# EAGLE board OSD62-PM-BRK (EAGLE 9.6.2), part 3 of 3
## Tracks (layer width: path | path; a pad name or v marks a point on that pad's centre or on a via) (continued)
VIN-5P0  (via drill 0.1 pad 0.25, 0.25 pad 0.46) (continued)
  pour Bottom: 86.23,5.97 86.23,7.75 84.71,7.75 84.71,5.97
  pour Bottom (no thermals): 64.52,16.89 65.79,16.89 65.79,17.53 65.28,18.03 64.52,18.03
  pour Top (no thermals): 64.52,18.03 65.28,18.03 65.79,17.53 65.79,16.89 64.52,16.89
  pour Bottom: 5.33,10.54 5.33,11.3 4.57,11.3 4.57,10.54
VMON_ER_SYS  (via drill 0.1 pad 0.25)
  Top 0.076: U1.A15 40.26,17.25 42.6,19.58 42.6,20.42 44.2,22.02 46.02,22.02 v46.18,22.17
  Top 0.127: R1.2 45.72,24.64 | 45.72,24.64 R2.1 | v45.72,24.31 45.72,24.64
  Bottom 0.076: v46.18,22.17 46.56,22.55 46.56,24.16 46.41,24.31 v45.72,24.31
VOUT0_DATA0  (via drill 0.1 pad 0.25)
  Top 0.076: U1.P26 v46,10.5
  Bottom 0.076: v46,10.5 46.37,10.5 46.56,10.31 46.56,7.01 48.23,5.33 49.99,5.33 50.67,4.65 50.67,2.67 JP2.21
VOUT0_DATA1  (via drill 0.1 pad 0.25)
  Top 0.076: U1.N25 v45.5,11
  Bottom 0.076: v45.5,11 45.75,10.75 46.35,10.75 46.71,10.39 46.71,7.09 48.31,5.49 50.44,5.49 52.07,3.86 JP3.21
VOUT0_DATA2  (via drill 0.1 pad 0.25)
  Top 0.076: U1.N26 v46,11
  Bottom 0.076: v46,11 46.33,11 47.32,10.01 47.32,6.71 48.39,5.64 52.27,5.64 53.19,4.72 53.19,2.69 JP2.22
VOUT0_DATA3  (via drill 0.1 pad 0.25)
  Top 0.076: U1.M25 v45.5,11.5
  Bottom 0.076: v45.5,11.5 45.75,11.25 46.31,11.25 47.47,10.09 47.47,6.78 48.46,5.79 52.65,5.79 54.61,3.83 JP3.22
VOUT0_DATA4  (via drill 0.1 pad 0.25)
  Top 0.076: U1.M26 v46,11.5
  Bottom 0.076: v46,11.5 46.29,11.5 47.62,10.16 47.62,6.86 48.54,5.94 54.63,5.94 55.7,4.88 55.7,2.72 JP2.23
VOUT0_DATA5
  Top 0.076: U1.U27 46.81,8.69 48.23,8.69 52.12,4.8 56.16,4.8 JP3.23
VOUT0_DATA6
  Top 0.076: U1.T27 46.5,9.5 47.65,9.5 52.2,4.95 57.61,4.95 58.29,4.27 58.29,2.67 JP2.24
VOUT0_DATA7
  Top 0.076: U1.T28 47.63,9.75 52.27,5.11 57.68,5.11 58.45,4.34 58.45,4.04 58.67,3.81 JP3.24
VOUT0_DATA8
  Top 0.076: U1.R27 46.5,10 47.61,10 52.35,5.26 57.76,5.26 58.22,4.8 60.2,4.8 60.81,4.19 60.81,2.69 JP2.25
VOUT0_DATA9
  Top 0.076: U1.R28 47.59,10.25 52.43,5.41 57.84,5.41 58.29,4.95 61.11,4.95 62.23,3.83 JP3.25
VOUT0_DATA10
  Top 0.076: U1.P27 46.5,10.5 47.56,10.5 52.5,5.56 57.91,5.56 58.37,5.11 62.64,5.11 63.32,4.42 63.32,2.72 JP2.26
VOUT0_DATA11
  Top 0.076: U1.P28 47.54,10.75 52.58,5.71 57.99,5.71 58.45,5.26 63.32,5.26 JP3.26
VOUT0_DATA12
  Top 0.076: U1.N27 46.5,11 47.52,11 52.65,5.87 58.06,5.87 58.52,5.41 64.92,5.41 65.84,4.5 65.84,2.74 JP2.27
VOUT0_DATA13
  Top 0.076: U1.N28 47.5,11.25 52.73,6.02 58.14,6.02 58.6,5.56 65.61,5.56 67.31,3.86 JP3.27
VOUT0_DATA14
  Top 0.076: U1.M27 46.5,11.5 47.48,11.5 52.81,6.17 58.22,6.17 58.67,5.71 67.36,5.71 68.43,4.65 68.43,2.69 JP2.28
VOUT0_DATA15
  Top 0.076: U1.M28 47.46,11.75 52.88,6.33 58.29,6.33 58.75,5.87 67.82,5.87 69.85,3.83 JP3.28
VOUT0_DE  (via drill 0.1 pad 0.25)
  Top 0.076: U1.R25 v45.5,10
  Bottom 0.076: v45.5,10 45.75,9.75 45.75,9.19 45.87,9.07 45.87,2.39 JP2.19
VOUT0_HSYNC  (via drill 0.1 pad 0.25)
  Top 0.076: U1.P25 v45.5,10.5
  Bottom 0.076: v45.5,10.5 45.75,10.25 46.17,10.25 46.41,10.01 46.41,6.93 JP3.20
VOUT0_PCLK  (via drill 0.1 pad 0.25)
  Top 0.076: U1.T26 v46,9.5
  Bottom 0.076: v46,9.5 46.02,9.47 46.02,4.72 46.94,3.81 JP3.19
VOUT0_VSYNC  (via drill 0.1 pad 0.25)
  Top 0.076: U1.R26 v46,10
  Bottom 0.076: v46,10 v46.01,10 46.25,9.75 46.25,6.71 48.39,4.57 48.39,2.41 JP2.20
VPP  (via drill 0.1 pad 0.25)
  Top 0.152: U1.C16 v41,16.5
  Bottom 0.254: v41,16.5 41.15,16.65 41.15,22.99 41.6,23.44 v41.6,24.08
  pour Top (no thermals): 41.25,25.02 41.25,23.57 41.45,23.37 42.04,23.37 42.04,25.02
VPP_EN
  Top 0.076: U14.3 40.65,22.73 J1.2 38.15,23.57 R3.2
WKUP_CLKOUT0  (via drill 0.1 pad 0.25)
  Top 0.076: U1.C7 v36,16.5 | v36.04,22.78 35.89,22.63 35.89,18.14 v36.12,17.91
  Bottom 0.076: v36.12,17.91 36,17.79 v36,16.5 | v36.04,22.78 36.27,23.01 36.27,24.77 35.89,25.15 35.89,28.27 JP5.15
WKUP_I2C0_SCL  (via drill 0.1 pad 0.25)
  Top 0.076: U1.A8 36.75,17.89 36.2,18.44 36.2,22.33 37.03,23.16 37.03,25.22 37.34,25.53 43.2,25.53 v43.59,25.15 | v46.63,19.43 46.94,19.13 49.99,19.13 57.15,11.96 70.33,11.96 71.09,11.2 71.09,9.46 J4.13 71.04,8.44 71.32,8.15 76.5,8.15 76.99,8.64 R64.1
  Bottom 0.076: v46.63,19.43 47.02,19.81 47.02,24.46 46.56,24.92 43.81,24.92 v43.59,25.15
WKUP_I2C0_SDA  (via drill 0.1 pad 0.25)
  Top 0.076: U1.B8 36.5,17 36.5,17.91 36.04,18.36 36.04,22.4 36.88,23.24 36.88,25.3 37.26,25.68 43.43,25.68 v43.59,25.53 | v47.02,19.43 47.17,19.28 50.06,19.28 57.23,12.12 71.32,12.12 72.01,11.43 72.01,9.44 J4.14 72.04,8.43 72.16,8.31 76.43,8.31 77.78,9.65 R12.1
  Bottom 0.076: v47.02,19.43 47.17,19.58 47.17,24.54 46.63,25.07 44.04,25.07 v43.59,25.53
WKUP_LFOSC0_XI
  Top 0.076: U1.H1 32.88,13.75 31.09,15.54 31.09,18.44 30.94,18.59 30.11,18.59 Y1.3
WKUP_UART0_CTSN
  Top 0.076: U1.D1 32.75,15.75 32.23,16.27 32.23,21.49 31.7,22.02 25.3,22.02 22.25,25.07 20.8,25.07 20.12,25.76 20.12,27.58 19.74,27.96 17.83,27.96 17.53,28.27 16,28.27 15.06,29.21 JP5.6
WKUP_UART0_RTSN
  Top 0.076: U1.D2 33.5,16 32.75,16 32.38,16.36 32.38,21.57 31.77,22.17 25.38,22.17 22.33,25.22 20.88,25.22 20.27,25.83 20.27,27.74 19.89,28.12 18.67,28.12 17.58,29.21 JP5.7
WKUP_UART0_RXD
  Top 0.076: U1.C2 33.5,16.5 32.88,16.5 32.69,16.69 32.69,21.72 31.93,22.48 25.53,22.48 22.48,25.53 21.03,25.53 20.57,25.98 20.57,28.19 JP5.9
WKUP_UART0_TXD
  Top 0.076: U1.C1 32.75,16.25 32.54,16.46 32.54,21.64 31.85,22.33 25.45,22.33 22.4,25.38 20.95,25.38 20.42,25.91 20.42,27.89 19.1,29.21 JP5.8

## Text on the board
tPlace: 10 | 20 | 30 | U0 | G | RX | TX | USB-C | PWR | VPP | JTAG | Rev 1D | 0 | 1 | 2 | 3 | PWR | CAMERA | 30 | 10 | OSD62-PM-BRK | 20 | 40
bPlace: GND | 5V | GND | 10 | 20 | 30 | GND | 3V3 | GND | GND | I2C Pull Ups / Solder if Needed | GND | 1V8 | Row D | GND | WP | SDA | SCL | JTAG | Row C | I2C0 | PORZ | STATZ | LVDS | ERRORN | 1 | 40 | TS_RESET | TS_INT# | Row B | I2C Pull Ups / Solder if Needed | GND | Row A | GND | 5V | 3V3 | 3V3 | 10 | 20 | 30 | GND | 5V | GND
